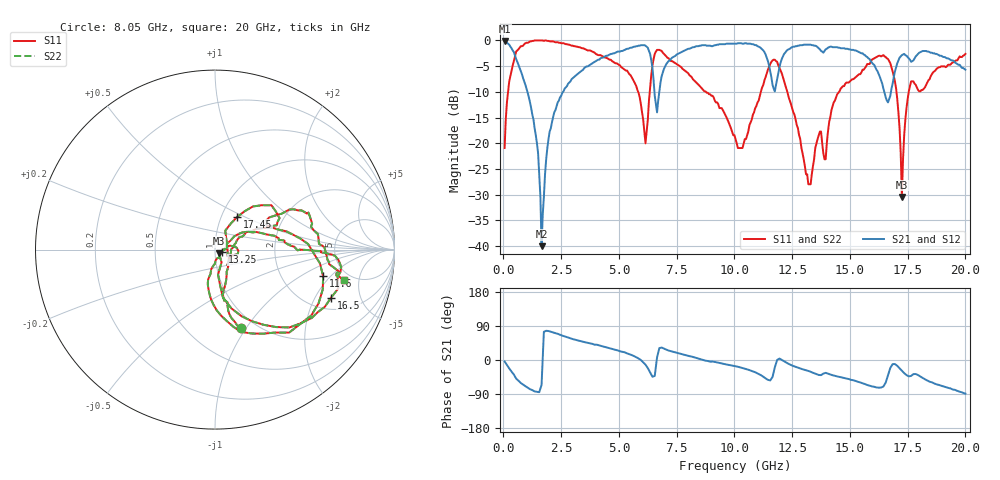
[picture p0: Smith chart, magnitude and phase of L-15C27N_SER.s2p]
# MHZ S MA R 50
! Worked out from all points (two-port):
!   400 points, 50 MHz to 20 GHz, reference 50 ohm
!   highest |S21| = -0.09 dB at 50 MHz (marker M1); lowest = -40.0 dB at 1.65 GHz (marker M2)
!   |S21| within 3 dB of the highest: 7.404 GHz to 11.38 GHz (3.974 GHz wide, 42.3 % of centre); 12.1 GHz to 15.7 GHz (3.597 GHz wide, 25.9 % of centre)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
!   lowest |S11| = -30.5 dB at 17.25 GHz (marker M3), VSWR 1.06, Z = 52.2 - j2.12 ohm
!   |S11| at or under -10 dB: 5.834 GHz to 6.333 GHz (498.8 MHz wide, 8.2 % of centre); 8.769 GHz to 11.14 GHz (2.375 GHz wide, 23.9 % of centre); 12.29 GHz to 14.53 GHz (2.242 GHz wide, 16.7 % of centre)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
!   |S22| runs from -30.5 to 0.0 dB; largest |S21 - S12| = 0
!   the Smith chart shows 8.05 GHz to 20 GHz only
!   S11 on the Smith chart (normalised r, x): 8.05 GHz: 0.85, -0.95; 11.6 GHz: 3.42, -1.64; 13.25 GHz: 1.08, -0.03; 16.5 GHz: 2.59, -2.73; 17.45 GHz: 1.19, +0.45; 20 GHz: 4.22, -3.17
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50  0.09 77.4  0.99 -3.8  0.99 -3.8  0.09 77.4
550  0.78 44.9  0.66 -49.0  0.66 -49.0  0.78 44.9
1300  0.99 11.4  0.17 -81.2  0.17 -81.2  0.99 11.4
1650  1 -0.4  0.01 -65.9  0.01 -65.9  1 -0.4
2000  0.98 -11.0  0.13 75.6  0.13 75.6  0.98 -11.0
3400  0.84 -41.8  0.51 48.9  0.51 48.9  0.84 -41.8
5500  0.46 -78.4  0.85 14.3  0.85 14.3  0.46 -78.4
6150  0.1 -42.9  0.89 -12.3  0.89 -12.3  0.1 -42.9
6700  0.81 -24.2  0.26 19.2  0.26 19.2  0.81 -24.2
8050  0.46 -71.7  0.83 10.1  0.83 10.1  0.46 -71.7
10050  0.11 -51.2  0.93 -16.6  0.93 -16.6  0.11 -51.2
11600  0.62 -13.8  0.44 -49.3  0.44 -49.3  0.62 -13.8
11950  0.54 -60.2  0.55 3.8  0.55 3.8  0.54 -60.2
13250  0.04 -18.3  0.91 -29.8  0.91 -29.8  0.04 -18.3
13350  0.05 0.9  0.9 -32.5  0.9 -32.5  0.05 0.9
14450  0.3 16.3  0.86 -43.6  0.86 -43.6  0.3 16.3
16500  0.7 -22.5  0.31 -64.7  0.31 -64.7  0.7 -22.5
16700  0.63 -40.7  0.27 -30.6  0.27 -30.6  0.63 -40.7
17050  0.27 -80.6  0.6 -15.4  0.6 -15.4  0.27 -80.6
17250  0.03 -42.6  0.72 -28.3  0.72 -28.3  0.03 -42.6
17450  0.22 55.9  0.71 -39.8  0.71 -39.8  0.22 55.9
20000  0.74 -13.3  0.52 -88.8  0.52 -88.8  0.74 -13.3
